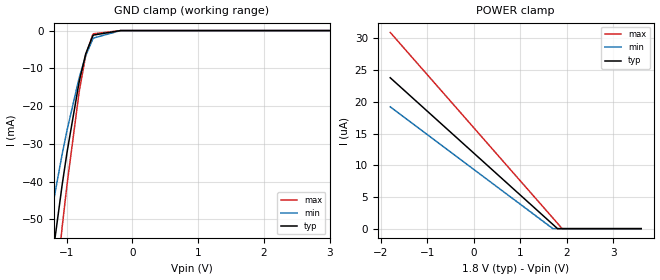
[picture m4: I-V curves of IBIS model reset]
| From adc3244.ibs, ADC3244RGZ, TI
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|   reset Model
[Model]   reset
Model_type   Input
Vinl = 0.4
Vinh = 1.2
|   typ   min   max
|   (nom PVT)   (fast PVT)   (slow PVT)
C_comp   1.280e-12   1.241e-12   1.322e-12
| Where nom  PVT is Nominal Process, 1.8V, 27C
|   Fast PVT is Strong Process,  1.9V, -40C
|   Slow PVT is Weak Process,   1.7V, 125C
[Voltage Range]   1.8   1.7   1.9
|Junction Temperature
[Temperature Range]   27   125   -40
[Power Clamp Reference]   1.8   1.7   1.9
[GND Clamp Reference]   0   0   0
[GND Clamp]
|   Voltage   I(typ)   I(min)   I(max)
-1.8V     -793mA     -162.7mA   -1.722A
-1.368V   -79.7mA    -61.08mA   -101.5mA
-1.069V   -40.85mA   -32.73mA   -52.01mA
-994.2mV  -32.2mA    -26.4mA    -40.74mA
-813.6mV  -13.94mA   -12.78mA   -16.69mA
-802.1mV  -12.95mA   -12.03mA   -15.4mA
-710.3mV  -6.162mA   -6.635mA   -6.578mA
-604.9mV  -1.494mA   -2.336mA   -1.139mA
-592.2mV  -1.188mA   -1.985mA   -852.4uA
-180mV    -1.194uA   -1.226uA   -1.505uA
3.6V      0A         0A         0A
[POWER Clamp]
|   Voltage   I(typ)   I(min)   I(max)
-1.8V     23.79uA    19.2uA     30.94uA
1.699V    670nA      0A         1.684uA
1.798V    11.89nA    0A         851.2nA
1.899V    0A         0A         0A
3.6V      0A         0A         0A
